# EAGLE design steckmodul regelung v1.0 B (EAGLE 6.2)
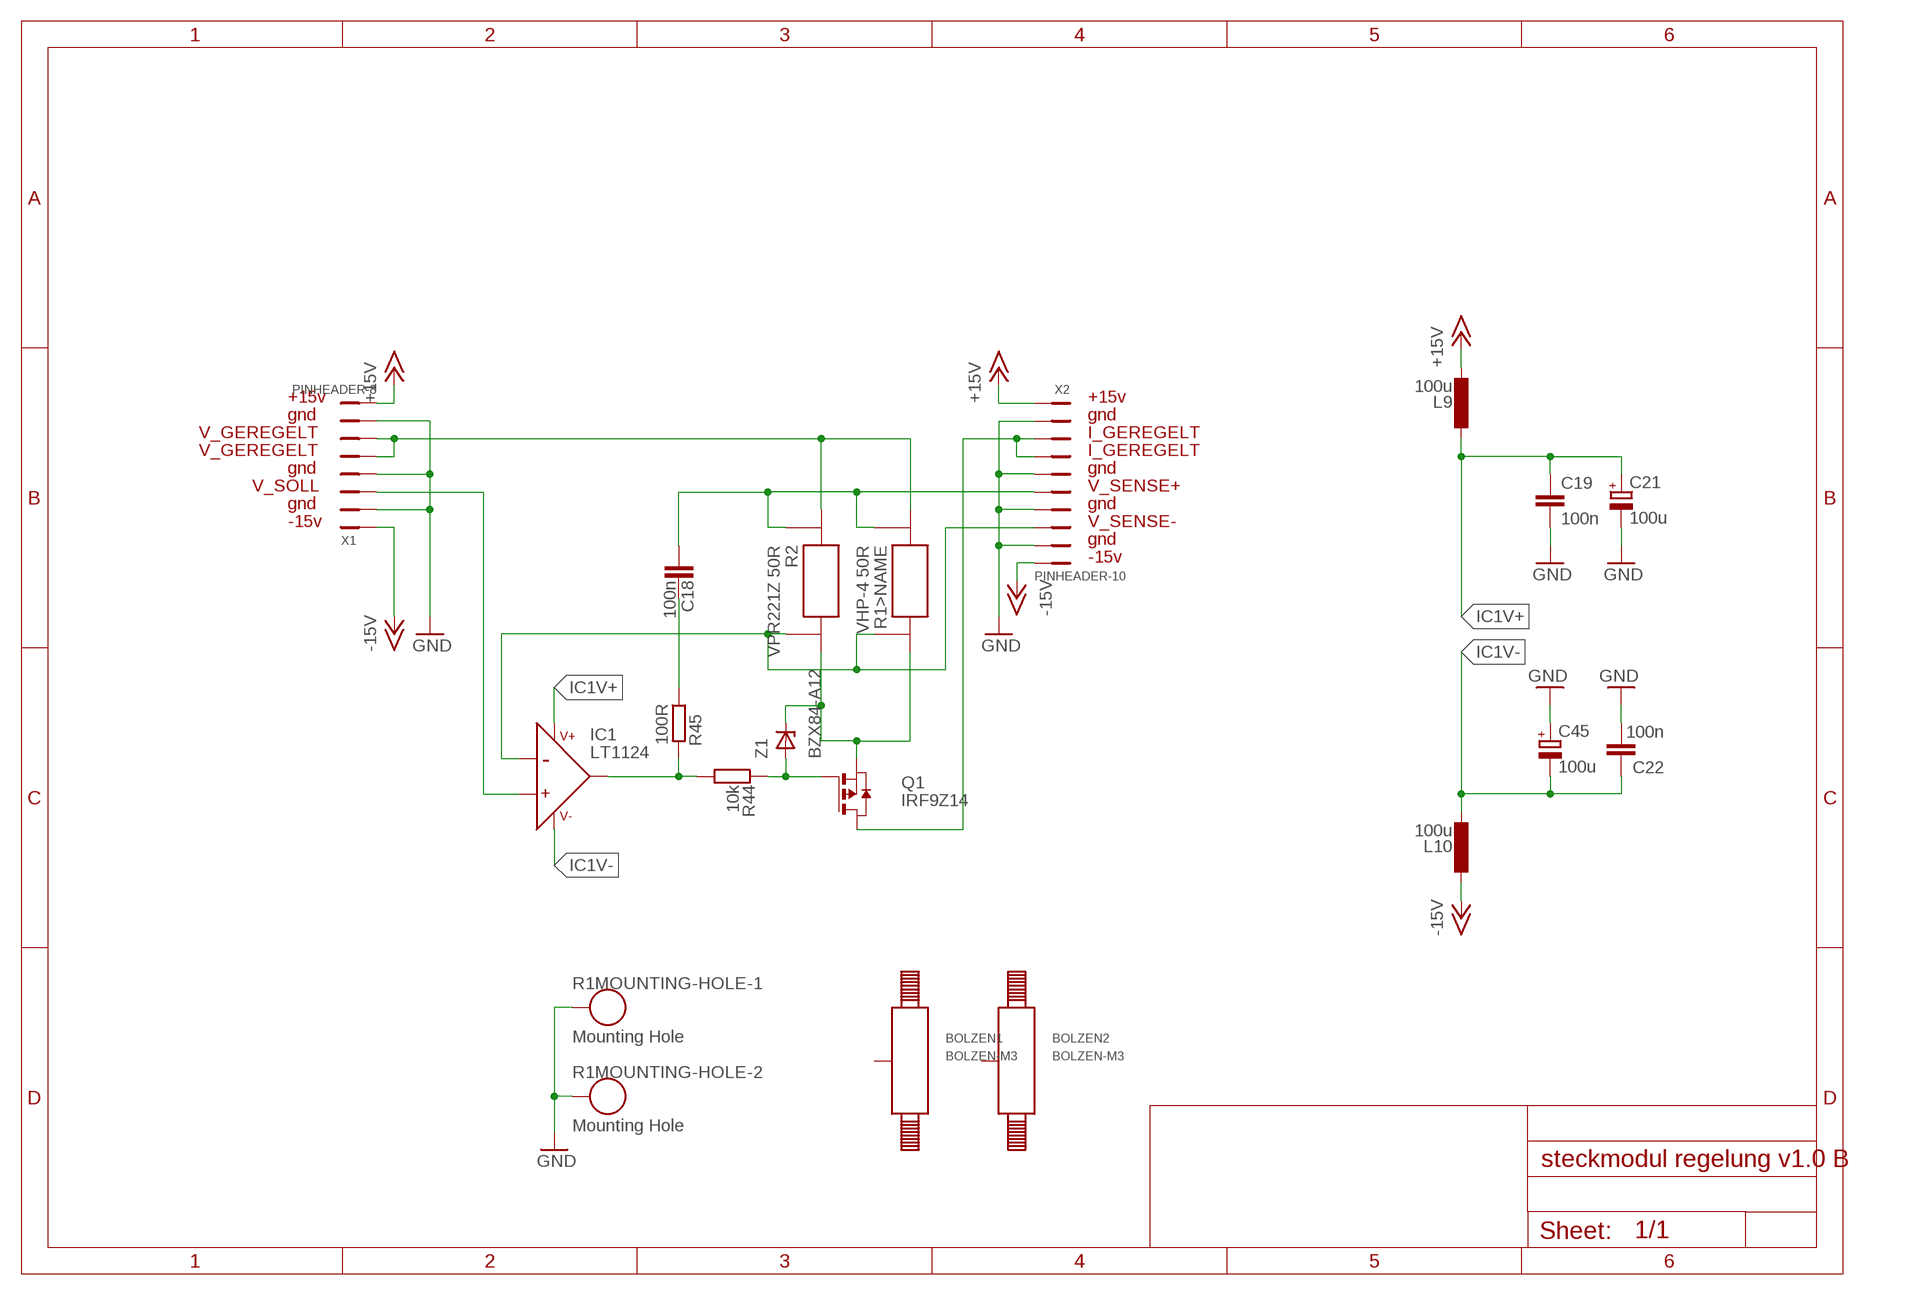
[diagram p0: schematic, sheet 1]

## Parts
BOLZEN1  BOLZEN-M3  [LOCH-M3]
BOLZEN2  BOLZEN-M3  [LOCH-M3]
C18  100n  C0805  [C0805]
C19  100n  C0805  [C0805]
C21  100u  C-POL100UF  [TT5D7]
C22  100n  C0805  [C0805]
C45  100u  C-POL100UF  [TT5D7]
IC1  LT1124  [S8]
L9  100u  L100MA100UH  [L-KLEIN]
L10  100u  L100MA100UH  [L-KLEIN]
Q1  IRF9Z14  [TO220]
R1  VHP-4 50R  VHP-4  [TO3-4]
R2  VPR221Z 50R  VPR221Z  [TO220-4]
R44  10k  R0805  [R0805]
R45  100R  R0805  [R0805]
X1  PINHEADER-8  [PINHEADER-8]
X2  PINHEADER-10  [PINHEADER-10]
Z1  BZX84-A12  BZX84  [SOT23]

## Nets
+15V: L9.2 X1.8 X2.1
-15V: L10.1 X1.1 X2.10
GND: C19.2 C21.- C22.2 C45.+ R1.5 R1.TO3/5 X1.2 X1.4 X1.7 X2.2 X2.5 X2.7 X2.9
IC1V+: C19.1 C21.+ IC1.6(V+) L9.1
IC1V-: C22.1 C45.- IC1.2(V-) L10.2
N$1: C18.2 R1.E1(>NAME:E1) R2.E1 X2.6
N$3: Q1.3(S) R1.I2(>NAME:I2) R2.I2 Z1.3(K)
N$4: IC1.8(-IN) R1.E2(>NAME:E2) R2.E2 X2.8
N$15: C18.1 R45.1
N$63: Q1.1(G) R44.1 Z1.1(A)
N$69: IC1.1(+IN) X1.3
N$75: IC1.7(OUT) R44.2 R45.2
N$76: Q1.2(D) X2.3 X2.4
N$146: R1.I1(>NAME:I1) R2.I1 X1.5 X1.6
Unconnected: BOLZEN1.1 BOLZEN2.1

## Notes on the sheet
- +15v | +15v
- gnd | gnd
- V_GEREGELT | I_GEREGELT
- V_GEREGELT | I_GEREGELT
- gnd | gnd
- V_SOLL | V_SENSE+
- gnd | gnd
- -15v | V_SENSE-
- gnd
- -15v

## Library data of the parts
BOLZEN1 BOLZEN2 = lasertreiber:BOLZEN
C18 C19 C22 = lasertreiber:C: Keramik- und Folienkondesatoren für Lasertreiber
C21 C45 = lasertreiber:C-POL: Polare Kondensatoren für den Lasertreiber
IC1 = lasertreiber:LT1124
L9 L10 = lasertreiber:L
Q1 = lasertreiber:IRF9Z14
R1 = lasertreiber:VHP-4
R2 = lasertreiber:VPR221Z
R44 R45 = lasertreiber:R
X1 = lasertreiber:PINHEADER-8
X2 = lasertreiber:PINHEADER-10
Z1 = lasertreiber:BZX84

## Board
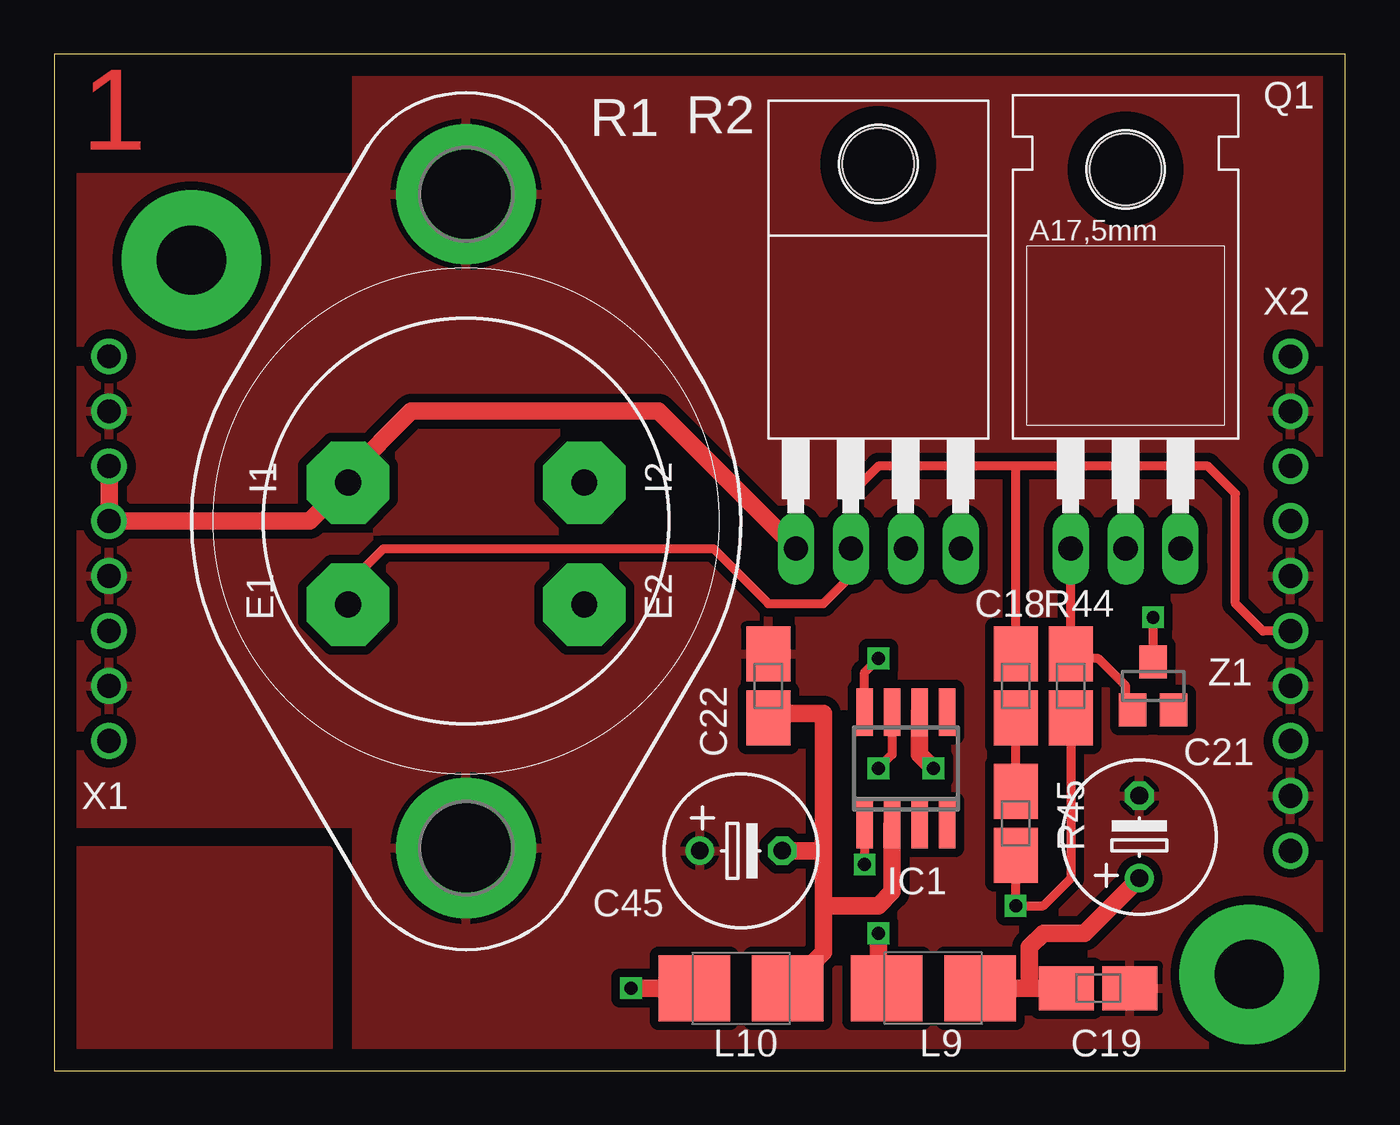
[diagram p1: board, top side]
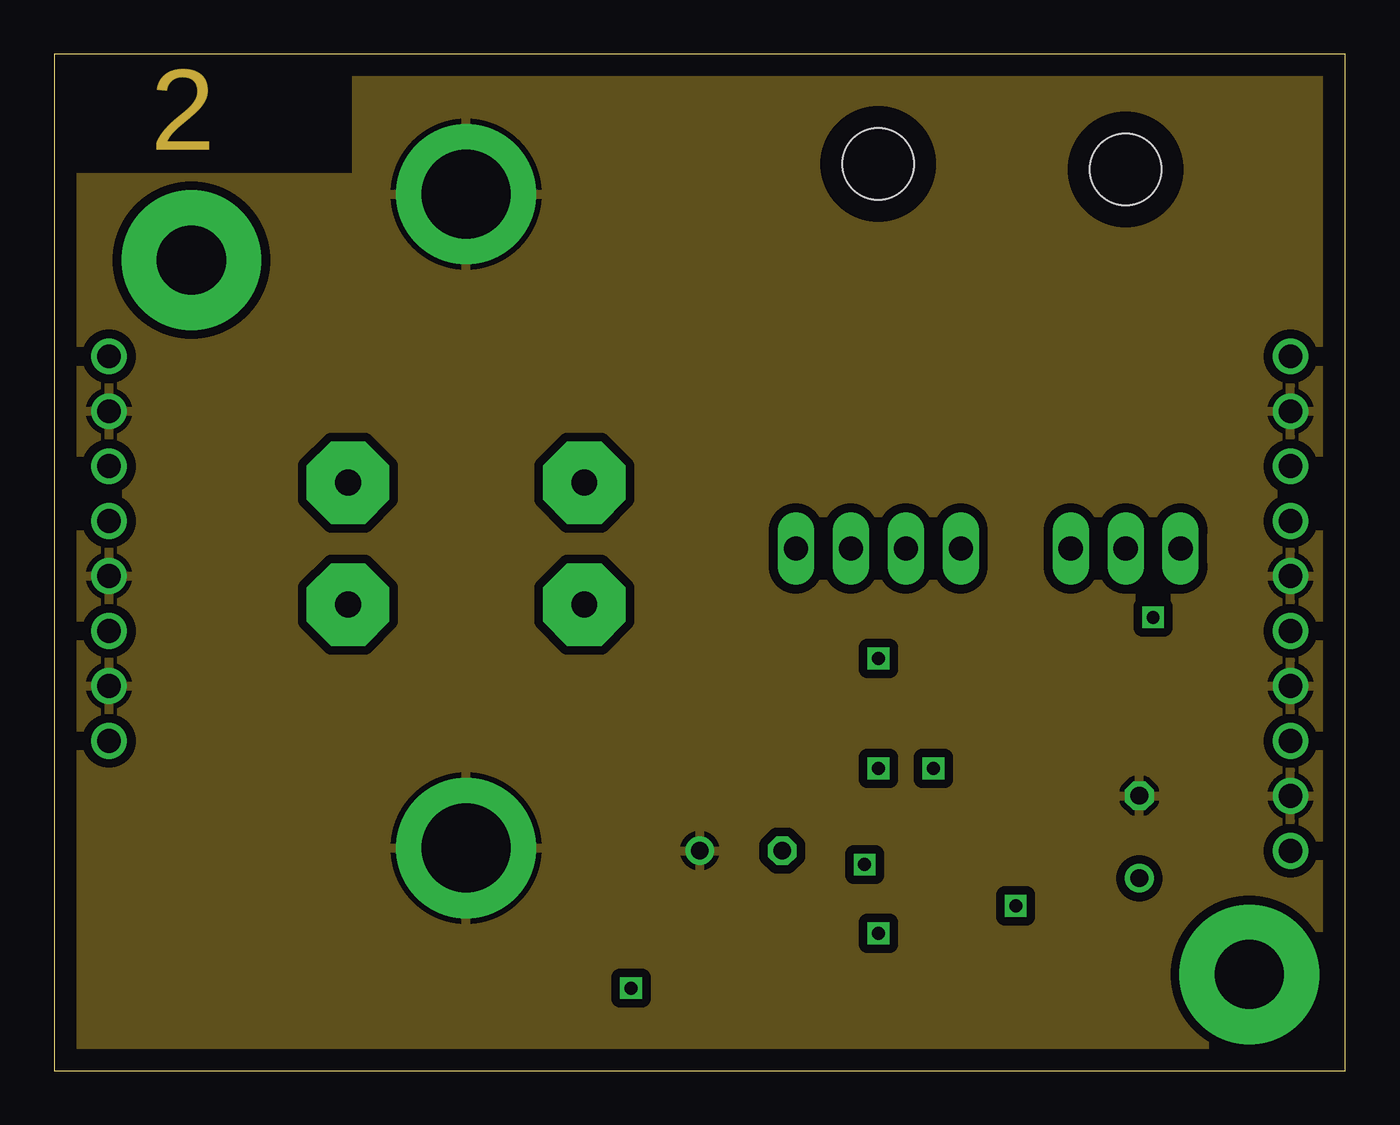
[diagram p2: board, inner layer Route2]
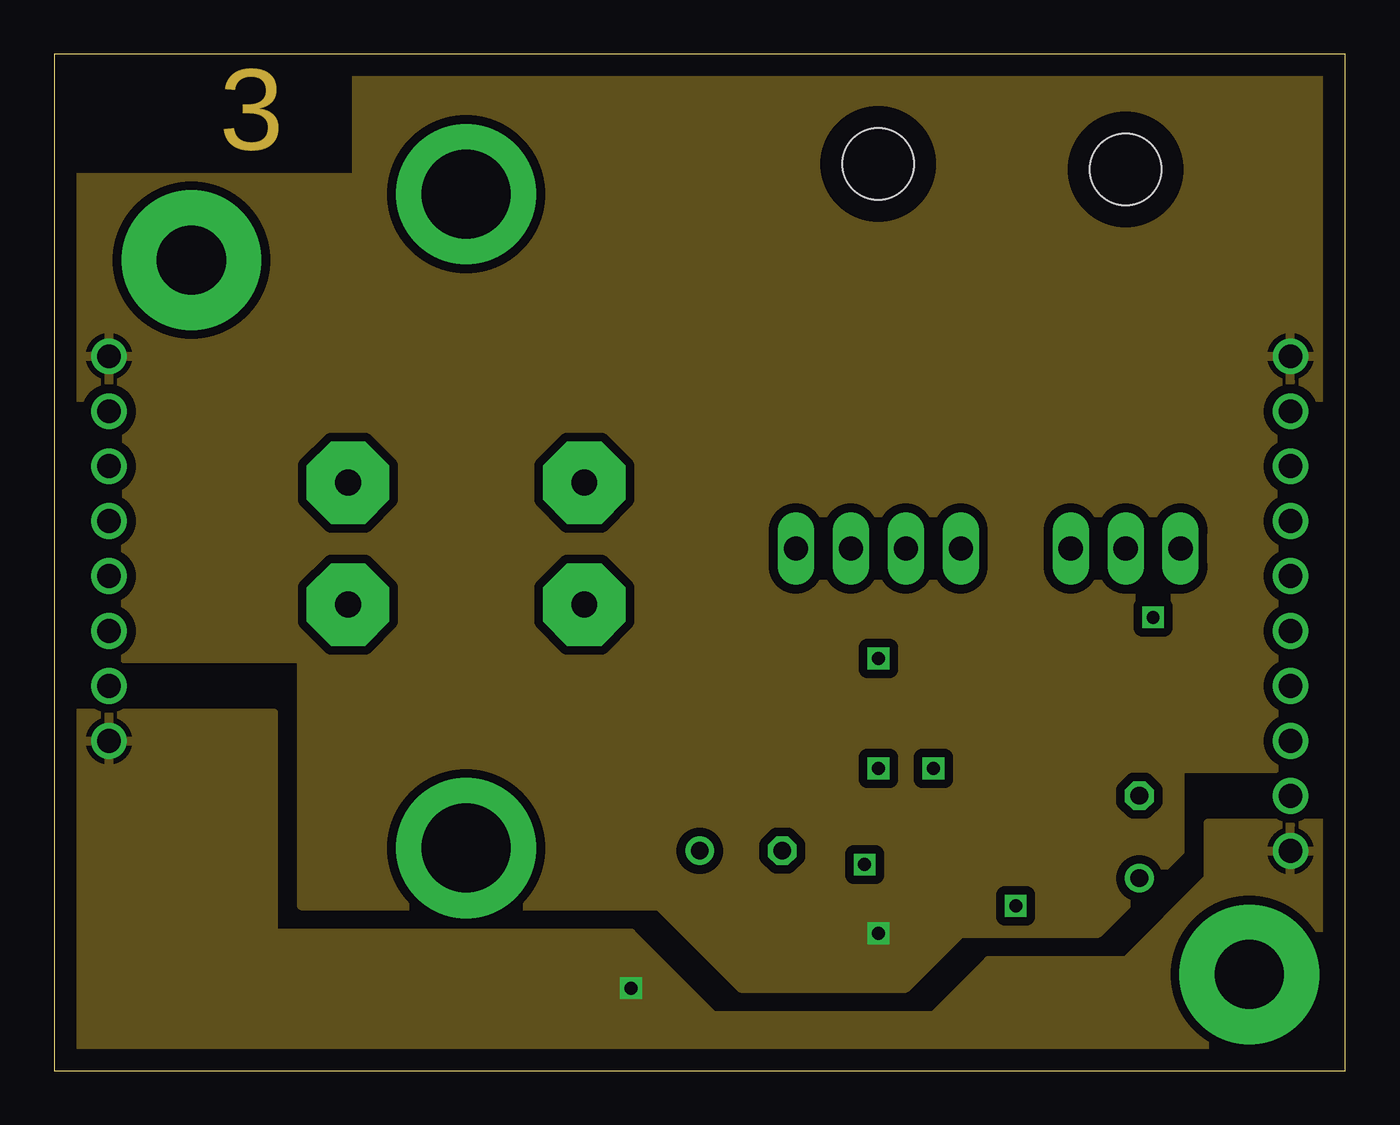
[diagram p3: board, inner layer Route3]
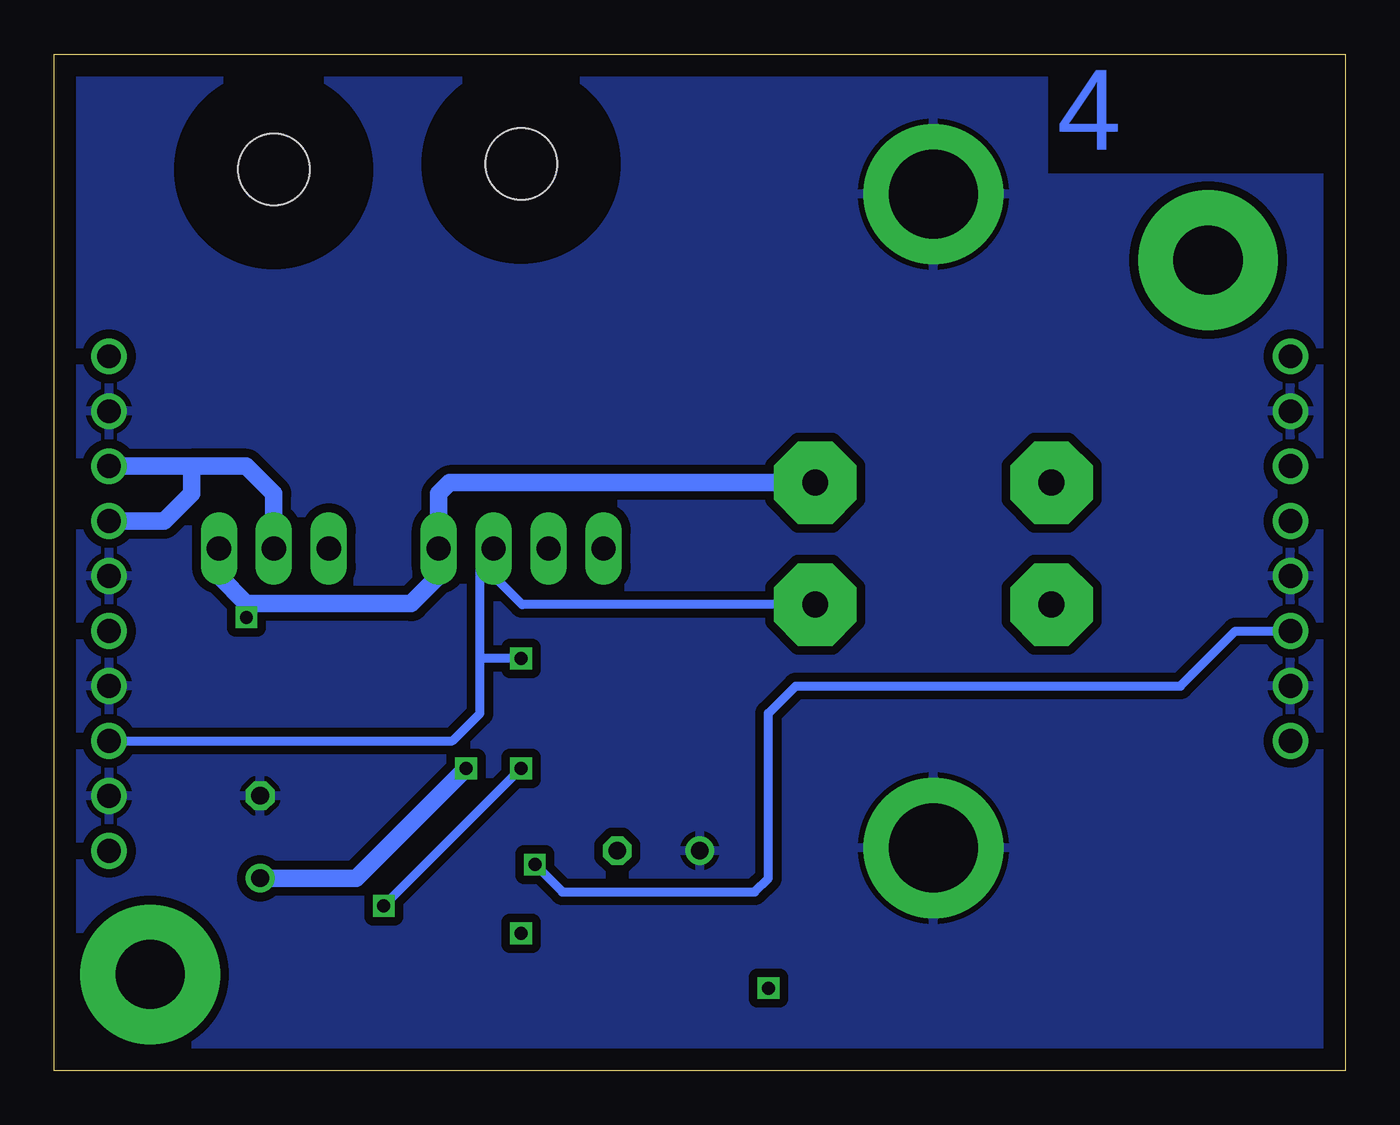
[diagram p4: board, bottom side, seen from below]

Size 59.69 x 46.99 mm. Coordinates in mm from the lower left corner, seen from the top.
Outline: 0,0 59.69,0 59.69,46.99 0,46.99 0,0
Copper layers (1+2*3+16): Top 0.018mm / dielectric 0.14mm / Route2 0.035mm / dielectric 1.2mm / Route3 0.035mm / dielectric 0.14mm / Bottom 0.018mm
Design rules: minimum track width 10mil, minimum drill 23mil, track to track 8mil, track to pad 8mil, pad to pad 8mil, via to via 8mil, smd to smd 8mil, copper to edge 40mil, drill to drill 8mil, minimum pad ring 10mil, minimum via ring 8mil, stop-mask expansion 4mil, vias tented up to drill 0mil, thermal gap 10mil

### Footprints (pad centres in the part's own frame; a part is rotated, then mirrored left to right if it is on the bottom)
LOCH-M3 = drill 3.2 pad 6.452: 1 0,0
C0805 = smd 2.54 x 2.032: 1 -1.473,0; 2 1.473,0
TT5D7 = drill 0.813: + -1.905,0 | drill 0.813 octagon: - 1.905,0
S8 = smd 0.762 x 2.2: 1 -1.905,-2.6; 2 -0.635,-2.6; 3 0.635,-2.6; 4 1.905,-2.6; 5 1.905,2.6; 6 0.635,2.6; 7 -0.635,2.6; 8 -1.905,2.6
L-KLEIN = smd 3.302 x 3.048: 1 -2.159,0; 2 2.159,0
TO220 = drill 1.118 long: 1 -2.54,-6.35; 2 0,-6.35; 3 2.54,-6.35 | hole 3.302: 0,11.176
TO3-4 = drill 4.115 pad 6.477: 5 15.113,0; TO3/5 -15.113,0 | drill 1.194 pad 3.81 octagon: E1 -3.861,5.461; E2 -3.861,-5.461; I1 1.778,5.461; I2 1.778,-5.461
TO220-4 = drill 1.118 long: E1 -1.27,-10.16; E2 1.27,-10.16; I1 -3.81,-10.16; I2 3.81,-10.16 | hole 3.302: 0,7.62
R0805 = smd 2.54 x 2.032: 1 -1.473,0; 2 1.473,0
PINHEADER-8 = drill 1.1: 1 -8.89,0; 2 -6.35,0; 3 -3.81,0; 4 -1.27,0; 5 1.27,0; 6 3.81,0; 7 6.35,0; 8 8.89,0
PINHEADER-10 = drill 1.1: 1 -11.43,0; 2 -8.89,0; 3 -6.35,0; 4 -3.81,0; 5 -1.27,0; 6 1.27,0; 7 3.81,0; 8 6.35,0; 9 8.89,0; 10 11.43,0
SOT23 = smd 1.27 x 1.524: 1 -0.95,-1.1; 2 0.95,-1.1; 3 0,1.1

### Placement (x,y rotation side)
BOLZEN1  55.24,4.45 0 top
BOLZEN2  6.35,37.47 0 top
C18  44.45,17.78 90 top
C19  48.26,3.81 0 top
C21  50.16,10.79 90 top
C22  33.02,17.78 90 top
C45  31.75,10.16 0 top
IC1  39.37,13.97 0 top
L9  40.64,3.81 180 top
L10  31.75,3.81 0 top
Q1  49.53,30.48 0 top
R1  19.05,25.4 90 top
R2  38.1,34.29 0 top
R44  46.99,17.78 270 top
R45  44.45,11.43 270 top
X1  2.54,24.13 90 top
X2  57.15,21.59 270 top
Z1  50.8,17.78 0 top

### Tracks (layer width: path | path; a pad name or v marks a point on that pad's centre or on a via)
+15V  (via drill 0.6)
  Top 0.406: L9.2 38.1,4.19
  Top 0.813: 38.1,4.19 v38.1,6.35
  pour Route3 (isolate 0.406, rank 2): 39.37,3.81 41.91,6.35 48.26,6.35 52.07,10.16 52.07,13.97 59.69,13.97 59.69,46.99 13.97,46.99 13.97,41.27 0,41.27 0,19.05 11.43,19.05 11.43,7.62 27.94,7.62 31.75,3.81
-15V  (via drill 0.6)
  Top 0.813: L10.1 v26.67,3.81
  pour Route3 (isolate 0.406): 0,0 59.69,0 59.69,11.43 53.34,11.43 53.34,8.89 49.53,5.08 43.18,5.08 40.64,2.54 30.48,2.54 26.67,6.35 10.16,6.35 10.16,16.51 0,16.51
GND
  pour Top (isolate 0.406): 0,41.27 0,11.43 13.97,11.43 13.97,0 59.69,0 59.69,46.99 13.97,46.99 13.97,41.27
  pour Bottom (isolate 0.406): 0,41.27 0,0 59.69,0 59.69,46.99 13.97,46.99 13.97,41.27
  pour Route2 (isolate 0.406): 0,41.27 0,0 59.69,0 59.69,46.99 13.97,46.99 13.97,41.27
IC1V+  (via drill 0.6)
  Top 0.813: L9.1 45.09,3.81 | 45.09,3.81 C19.1 | 45.09,3.81 45.09,5.71 45.72,6.35 47.62,6.35 C21.+ | IC1.6 40.01,14.61 v40.64,13.97
  Bottom 0.813: C21.+ 45.72,8.89 v40.64,13.97
IC1V-
  Top 0.813: 35.56,7.62 35.56,5.46 L10.2 | 35.56,7.62 35.56,10.16 | 35.56,10.16 35.56,16.51 33.22,16.51 C22.1 | C45.- 35.56,10.16 | IC1.2 38.73,8.26 38.1,7.62 35.56,7.62
N$1
  Top 0.406: R1.E1 13.59,22.48 15.24,24.13 30.48,24.13 33.02,21.59 35.56,21.59 36.83,22.86 R2.E1 36.83,26.67 38.1,27.94 44.45,27.94 | C18.2 44.45,27.94 | 44.45,27.94 53.34,27.94 54.61,26.67 54.61,21.59 55.88,20.32 X2.6
N$2
  pour Top: 0,10.16 0,0 12.7,0 12.7,10.16
N$3  (via drill 0.6)
  Top 0.406: Z1.3 v50.8,20.95
  Bottom 0.406: R2.I2 41.91,22.86 | v50.8,20.95 50.8,21.59
  Bottom 0.813: R1.I2 41.4,27.18 41.91,26.67 R2.I2 | 41.91,22.86 43.18,21.59 50.8,21.59 52.07,22.86 Q1.3
N$4  (via drill 0.6)
  Top 0.406: 40.01,23.5 R2.E2 | IC1.8 37.47,18.41 v38.1,19.05
  Bottom 0.406: R1.E2 38.05,21.54 39.37,22.86 R2.E2 40.01,23.5 40.01,19.05 | 40.01,19.05 40.01,16.51 41.27,15.24 X2.8 | v38.1,19.05 40.01,19.05
N$15
  Top 0.406: R45.1 C18.1
N$63
  Top 0.406: Q1.1 R44.1 47.19,19.05 48.26,19.05 49.53,17.78 49.53,16.68 Z1.1
N$69  (via drill 0.6)
  Top 0.406: v37.47,9.53 IC1.1 37.47,11.43
  Bottom 0.406: v37.47,9.53 36.2,8.26 27.3,8.26 26.67,8.89 26.67,16.51 25.4,17.78 7.62,17.78 5.08,20.32 X1.3
N$75  (via drill 0.6)
  Top 0.406: R44.2 46.99,8.89 45.72,7.62 v44.45,7.62 R45.2 | IC1.7 38.73,14.61 v38.1,13.97
  Bottom 0.406: v38.1,13.97 v44.45,7.62
N$76
  Bottom 0.813: Q1.2 49.53,26.67 50.8,27.94 53.34,27.94 | 53.34,27.94 53.34,26.67 54.61,25.4 X2.4 | X2.3 53.34,27.94
N$146
  Top 0.813: R2.I1 27.94,30.48 16.51,30.48 13.59,27.56 R1.I1 11.81,25.4 X1.5 X1.6

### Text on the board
Top: 1
Route2: 2
Route3: 3
Bottom: 4
tStop: Inst. f. Quantenoptik | LU Hannover | J.R. Holst, S. Sauer | Steckmodul B | 2021-01-18 | Version 1 | Serie 1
